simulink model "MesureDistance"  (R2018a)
settings: Solver=FixedStepAuto  StartTime=0.0  StopTime=inf  FixedStep=0.1  RelTol=1e-3  EnableMultiTasking=on
undefined symbols (not defined in the file): b9c4a659, d30d, de3bed5c, fd68, hex2dec, pushbutton, semicirculargauge, serial, Telemetre
libraries: instrumentlib x3, dspindex x1

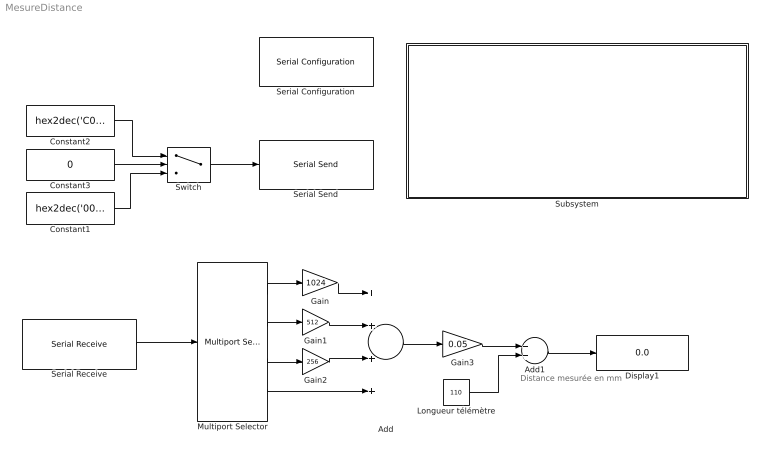
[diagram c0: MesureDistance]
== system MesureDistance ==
  note: Distance mesurée en mm
  Add : Sum  Inputs=++++
  Add1 : Sum
  Constant1 : Constant  Value=hex2dec('00')  OutDataTypeStr=uint32
  Constant2 : Constant  Value=hex2dec('C04000EE')  OutDataTypeStr=uint32
  Constant3 : Constant  Value=0  OutDataTypeStr=uint32
  Display1 : Display
  Gain : Gain  Gain=1024
  Gain1 : Gain  Gain=512
  Gain2 : Gain  Gain=256
  Gain3 : Gain  Gain=0.05
  Longueur télémètre : Constant  Value=110
  Multiport Selector : dspindex/Multiport Selector  rowsOrCols=Rows  idxCellArray={2,3,4,5}  idxErrMode=Clip Index
  Serial Configuration : instrumentlib/Serial Configuration  Priority=-200000  ComPortMenu=<Please select a port...>  ComPort=COM19  ObjConstructor=serial('COM19');  BaudRate=9600  DataBits=8  Parity=none  StopBits=1  FlowControl=none  Timeout=1  ByteOrder=BigEndian
  Serial Receive : instrumentlib/Serial Receive  ComPortMenu=<Please select a port...>  ComPort=COM19  ObjConstructor=serial('COM19');  Terminator=<none>  DataSize="[7  1]"  DataType=uint8  EnableBlockingMode=on  ActionDataUnavailable=Output last received value  CustomValue=0  SampleTime=0.1
  Serial Send : instrumentlib/Serial Send  ComPortMenu=<Please select a port...>  ComPort=COM19  ObjConstructor=serial('COM19');  Terminator=<none>  EnableBlockingMode=on
  Subsystem : Subsystem
  Switch : Switch  Criteria=u2 > Threshold
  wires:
  Switch/1 -> Serial Send/1
  Constant2/1 -> Switch/1
  Constant1/1 -> Switch/3
  Constant3/1 -> Switch/2
  Serial Receive/1 -> Multiport Selector/1
  Multiport Selector/2 -> Gain1/1
  Multiport Selector/3 -> Gain2/1
  Gain1/1 -> Add/2
  Gain2/1 -> Add/3
  Multiport Selector/4 -> Add/4
  Multiport Selector/1 -> Gain/1
  Add/1 -> Gain3/1
  Gain/1 -> Add/1
  Gain3/1 -> Add1/1
  Longueur télémètre/1 -> Add1/2
  Add1/1 -> Display1/1

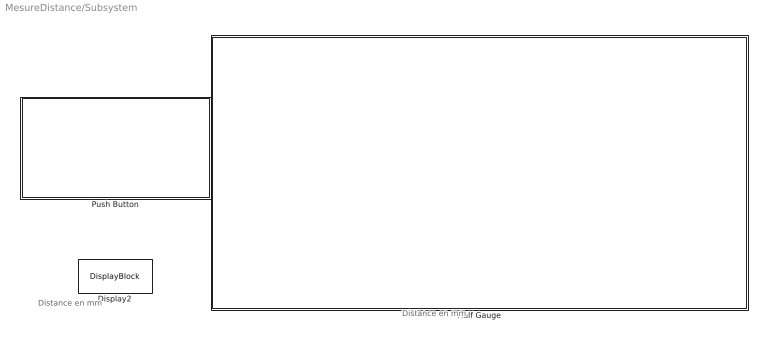
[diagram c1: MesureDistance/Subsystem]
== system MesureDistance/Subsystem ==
  note: Distance en mm
  note: Distance en mm
  Display2 : DisplayBlock  WebBlockId=99  LabelPosition=Hide
  Half Gauge : Subsystem  DialogController=hmiCreateDDGDialog  IsWebBlock=on  mask(MWDashboardBlock){webBlockId=de3bed5c-d30d-4207-9a71-35f502ca5a66, webBlockType=semicirculargauge, ShowInLibBrowser=on, ShowInitialText=on, HMISrcModelName=Telemetre}
      mask prompts: webBlockId "WebBlock Id"; webBlockType "WebBlock Type"; HMISrcModelName "Source Model"
      mask help: SimulinkHMI:dialogs:SemicircularGaugeDialogDesc
  Push Button : Subsystem  DialogController=hmiCreateDDGDialog  IsWebBlock=on  mask(MWDashboardBlock){webBlockId=b9c4a659-fd68-4c7c-9bd9-178d2e7dbfb2, webBlockType=pushbutton, ShowInLibBrwoser=on, ShowInitialText=on, HMISrcModelName=Telemetre}
      mask prompts: webBlockId "WebBlock Id"; webBlockType "WebBlock Type"; HMISrcModelName "Source Model"
      mask help: SimulinkHMI:dialogs:PushButtonDialogDesc

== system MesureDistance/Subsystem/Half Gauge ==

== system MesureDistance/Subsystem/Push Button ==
